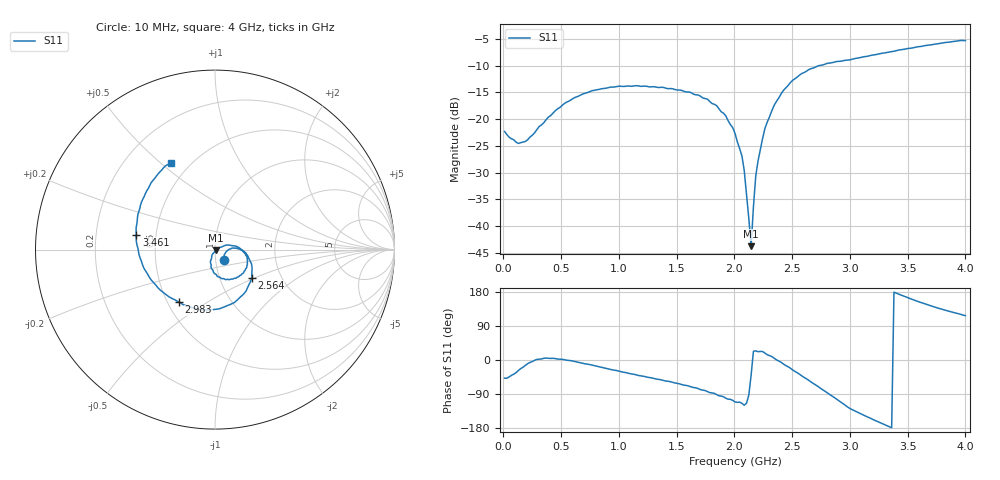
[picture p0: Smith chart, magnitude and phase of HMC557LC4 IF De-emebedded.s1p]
! Hittite Microwave Corporation
! 20 Alpha Road
! Chelmsford, MA 01824
! http://www.hittite.com
! Tel: 978-250-3343
! Fax: 978-250-3373
! Device:  HMC557LC4
! Description: GaAS MMIC Fundamental  Mixer
! Frequency:  2.5 -  7 GHz Mixer
! Package:  LC4  - Ceramic- 24 pins
! Ports:  1,IF Port De-emdedd from 10MHz - 5GH @ -10dBm,LO = 6GHz @ 15dBm, RF pORT Terminated  !
! Data:  The device was measured on evaluation board 118703.
!  The evaluation circuit board was modeled and simulated.  This was use
!  to removed the evaluation board circuit from the measured data.
!  The reference plane is the center of the package pin.
! Misc:
! Date Measured:  20-02-2008
! Date:  21-02-2008
! Note:
!  Hittite supplies this data as a sample of measured data at the package pin for
!  for this package product.  Your particular data for this product may vary.
!  Data was taken at 25 degrees C.
!  Hittite reserves the right to change this data at anytime.
# MHz S MA R 50
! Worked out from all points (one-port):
!   201 points, 10 MHz to 4 GHz, reference 50 ohm
!   lowest |S11| = -43.8 dB at 2.145 GHz (marker M1), VSWR 1.01, Z = 50.5 - j0.418 ohm
!   |S11| at or under -10 dB: start of sweep to 2.737 GHz
!   S11 on the Smith chart (normalised r, x): 10 MHz: 1.10, -0.13; 2.564 GHz: 1.42, -0.48; 2.983 GHz: 0.57, -0.38; 3.461 GHz: 0.39, +0.08; 4 GHz: 0.40, +0.54
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10  0.07648 -48.1
129.7  0.05911 -27.6
189.55  0.06168 -14.4
508.75  0.134 1.8
768.1  0.184 -13.5
1007.5  0.2031 -30.0
1506.25  0.1865 -61.6
1845.4  0.1336 -91.3
1925.2  0.107 -100.9
2005  0.07359 -110.6
2064.85  0.04525 -114.3
2084.8  0.03312 -119.3
2144.65  0.00648 -39.7
2164.6  0.0151 23.0
2184.55  0.02926 24.2
2204.5  0.04061 21.9
2264.35  0.08179 18.2
2344.15  0.1344 4.6
2503.75  0.2298 -26.0
2563.6  0.2575 -37.5
2803  0.3312 -86.3
2982.55  0.3555 -124.6
3002.5  0.3579 -128.4
3261.85  0.4092 -165.2
3461.35  0.4461 169.3
3501.25  0.4562 164.4
3800.5  0.5151 133.7
4000  0.5407 117.1
